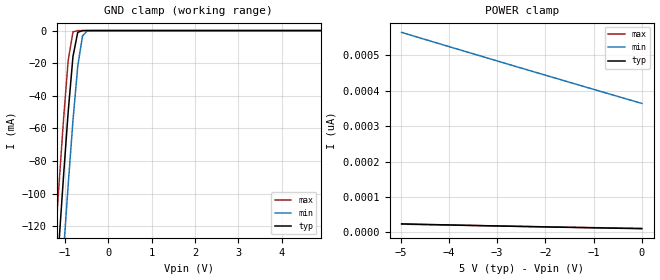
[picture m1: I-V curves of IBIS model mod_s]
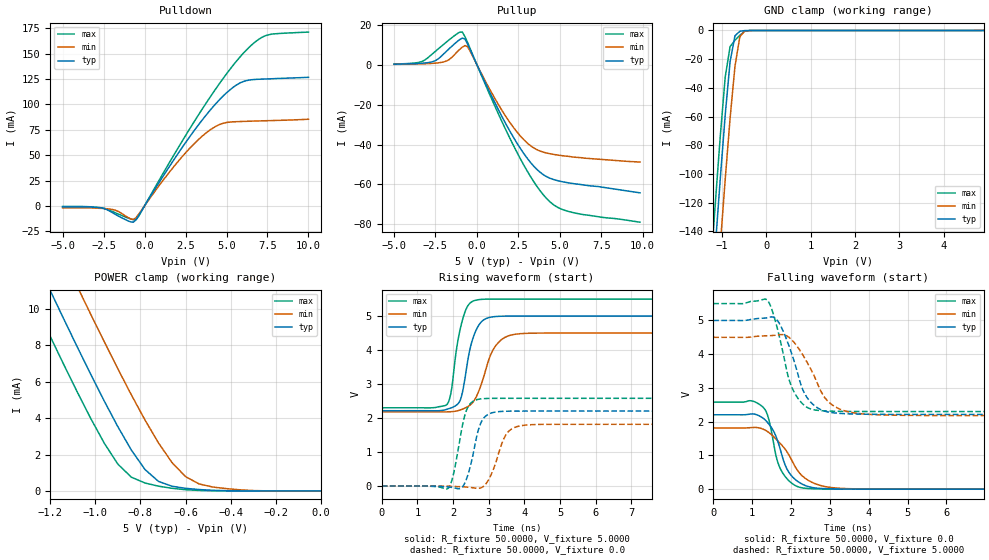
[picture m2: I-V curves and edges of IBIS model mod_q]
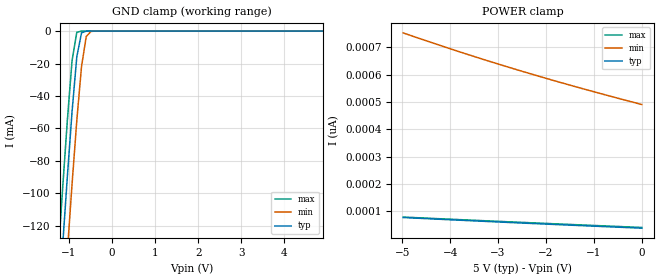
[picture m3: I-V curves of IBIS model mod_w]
| IBIS (I/O, Buffer, Information, Specification) Model, officially
| electronic behavioral standard for Buffer structures of digital pins.
[IBIS ver]  4.0
[File name] m95xxx_g12_tssop8.ibs
[File Rev]  1.0
[Date]   9 Oct 2015
[Source]   CAD & Design Services (Catania) - STMicroelectronics
[Notes]
  (Note1)  This IBIS model includes the TSSOP8 ceramic package parasitic data
  (Note2)  This IBIS model considers: VCC=5.0(TYP), 4.50(MIN), 5.50(MAX)
  (Note3)  This IBIS model has some Notes about the non-monotonicity
   of the I-V curves, but they are not indicative of problems
   inside the model;
[Copyright] (c) 2015 STMicroelectronics
|   Component M95XXX
[Component] M95XXX
[Manufacturer] STMicroelectronics
[Package]
|variable   typ   min   max
R_pkg   0.0   0.0   0.0
L_pkg   0.0H   0.0H   0.0H
C_pkg   0.0F   0.0F   0.0F
[Pin]   signal_name   model_name   R_pin   L_pin   C_pin
1   SN   mod_s   NA   NA   NA
2   Q   mod_q   NA   NA   NA
3   WN   mod_w   NA   NA   NA
4   GND   GND   NA   NA   NA
5   D   mod_s   NA   NA   NA
6   C   mod_s   NA   NA   NA
7   HOLDN   mod_h   NA   NA   NA
8   VCC   POWER   NA   NA   NA
[Package Model]  182696_TSSOP8
[Define Package Model]  182696_TSSOP8
[Manufacturer]  STMicroelectronics
[OEM]  STMicroelectronics
[Description]  8 pin TSSOP package
[Number Of Pins]  8
[Pin Numbers]
|Pin Num   Terminal Name
1   | net1
2   | net2
3   | net3
4   | net4_GND
5   | net5
6   | net6
7   | net7
8   | net8_VDD
[Model Data]
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[End Model Data]
[End Package Model]
| Models and submodels in the file (4): mod_s (Input), mod_q (I/O), mod_w (Input), mod_h (Input)
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|   Model mod_s
[Model]   mod_s
Model_type Input
Vinl   =   1.500V
Vinh   =   3.500V
C_comp   2.119pF   2.024pF   2.323pF
[Temperature Range]   25.0000   0.1050k   -40.0000
[Voltage Range]   5.0000V   4.5000V   5.5000V
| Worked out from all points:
|   GND clamp passes 1 mA (typ) near -0.70 V on its own axis
[GND_clamp]
|Voltage   I(typ)   I(min)   I(max)
-5V       -1.764A    -1.807A    -1.733A
-1.26V    -176.7mA   -223.6mA   -141.2mA
-1.15V    -132.7mA   -179.4mA   -97.27mA
-1.04V    -89.88mA   -136.2mA   -55.14mA
-930mV    -49.58mA   -94.31mA   -18.16mA
-820mV    -15.87mA   -55.06mA   -757uA
-710mV    -1.068mA   -21.8mA    -5.45uA
-600mV    -23.1uA    -3.301mA   -36.27nA
-490mV    -459.2nA   -183.8uA   -242.2pA
4.9V      10.56pA    379.5pA    10.13pA
[POWER_clamp]
|Voltage   I(typ)   I(min)   I(max)
-4.98V    24.27pA    563.8pA    23.46pA
-3.96V    21.17pA    522.2pA    20.77pA
-2.64V    17.45pA    468.9pA    17.5pA
0V        10.79pA    363.7pA    11.44pA
|   Model mod_q
[Model]   mod_q
Model_type I/O
Polarity   Non-Inverting
Enable   Active-Low
Vinl   =   1.500V
Vinh   =   3.500V
Vmeas  =   2.500V
Cref   =   30pF
C_comp   2.793pF   2.547pF   3.063pF
[Temperature Range]  25.0000   0.1050k   -40.0000
[Voltage Range]   5.0000V   4.5000V   5.5000V
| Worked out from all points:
|   slope of the pulldown table from 0 to 0.75 V, typ, clamps not added: 38.4 ohm
|   slope of the pullup table from 0 to 0.75 V, typ, clamps not added: 56.1 ohm
|   GND clamp passes 1 mA (typ) near -0.62 V on its own axis
|   POWER clamp passes 1 mA (typ) near -0.76 V on its own axis
|   rising waveform, R_fixture 50.0000, V_fixture 5.0000: 20-80 % time 324ps typ, 480ps min, 286ps max; typ from 2.21 V to 5 V
|   rising waveform, R_fixture 50.0000, V_fixture 0.0: 20-80 % time 297ps typ, 373ps min, 281ps max; typ from 0 V to 2.21 V
|   falling waveform, R_fixture 50.0000, V_fixture 0.0: 20-80 % time 452ps typ, 681ps min, 339ps max; typ from 2.21 V to 0 V
|   falling waveform, R_fixture 50.0000, V_fixture 5.0000: 20-80 % time 497ps typ, 646ps min, 427ps max; typ from 5 V to 2.21 V
[Pulldown]
|Voltage   I(typ)   I(min)   I(max)
-5V       -1mA       -2mA       -600uA
-2.6V     -2.1mA     -2.5mA     -2mA
-1.8V     -8.2mA     -4.2mA     -6.7mA
-840mV    -15.83mA   -12.84mA   -12.96mA
-520mV    -13.63mA   -11.72mA   -13.73mA
1.4V      35.96mA    30.85mA    39.51mA
3V        73.61mA    60.85mA    82.31mA
4.28V     99.55mA    77.79mA    113.9mA
5.24V     114.8mA    82.7mA     135.3mA
6.2V      123.5mA    83.38mA    153.5mA
7.32V     125.1mA    83.93mA    167.5mA
10V       126.8mA    85.45mA    171.4mA
[Pullup]
|Voltage   I(typ)   I(min)   I(max)
-5V       270uA      190uA      350uA
-3.44V    670uA      405uA      1.305mA
-2.64V    1.605mA    706uA      5.755mA
-1.68V    7.984mA    2.565mA    12.44mA
-880mV    13.35mA    8.83mA     16.36mA
-560mV    10.29mA    8.992mA    11.08mA
1.04V     -18.3mA    -16.27mA   -19.93mA
2.32V     -37.98mA   -32.67mA   -42.33mA
3.28V     -49.41mA   -40.84mA   -56.63mA
4.24V     -56.24mA   -44.29mA   -67.33mA
5.68V     -59.39mA   -46.1mA    -73.85mA
9.84V     -64.2mA    -48.78mA   -78.9mA
[GND_clamp]
|Voltage   I(typ)   I(min)   I(max)
-5V       -1.919A    -1.961A    -1.893A
-1.26V    -197.2mA   -244mA     -167mA
-1.15V    -149.4mA   -196.2mA   -119.1mA
-1.04V    -102.8mA   -149.2mA   -73.18mA
-930mV    -58.88mA   -103.8mA   -32.39mA
-820mV    -21.66mA   -61.22mA   -11.23mA
-710mV    -3.687mA   -24.94mA   -6.819mA
-600mV    -560.4uA   -4.331mA   -3.354mA
-490mV    -78.82uA   -439.8uA   -616.8uA
-380mV    -6.109uA   -68.67uA   -6.344uA
4.9V      210.5pA    105.8uA    176.1pA
[POWER_clamp]
|Voltage   I(typ)   I(min)   I(max)
-4.98V    114.4mA    117.5mA    112.1mA
-1.32V    14.15mA    17.49mA    11.63mA
-1.26V    12.57mA    15.9mA     10.05mA
-1.2V     10.99mA    14.33mA    8.479mA
-1.08V    7.9mA      11.22mA    5.424mA
-1.02V    6.392mA    9.687mA    3.968mA
-960mV    4.924mA    8.178mA    2.612mA
-840mV    2.238mA    5.266mA    752uA
-720mV    522.7uA    2.637mA    261.1uA
-600mV    143uA      786uA      68.21uA
-420mV    12.23uA    128uA      1.15uA
0V        225pA      1.615nA    241.5pA
[Ramp]
| variable   typ   min   max
dV/dt_r  1.3231/0.3352n   1.0895/0.4279n   1.5474/0.3147n
dV/dt_f  1.6706/0.5497n   1.3898/0.7138n   1.9193/0.4691n
R_load = 50.0000
[Rising Waveform]
R_fixture= 50.0000
V_fixture= 5.0000
V_fixture_min= 4.5000
V_fixture_max= 5.5000
|time   V(typ)   V(min)   V(max)
0s        2.215V     2.181V     2.301V
1.845ns   2.264V     2.181V     2.418V
1.935ns   2.293V     2.185V     2.703V
2.115ns   2.395V     2.21V      4.148V
2.265ns   2.761V     2.261V     4.888V
2.475ns   4.029V     2.379V     5.379V
2.655ns   4.602V     2.632V     5.471V
3.135ns   4.98V      4.027V     5.499V
3.735ns   5V         4.463V     5.5V
15ns      5V         4.5V       5.5V
[Rising Waveform]
R_fixture= 50.0000
V_fixture= 0.0
V_fixture_min= 0.0
V_fixture_max= 0.0
|time   V(typ)   V(min)   V(max)
0s        7.297nV    284nV      7.334nV
1.875ns   -26.33mV   -5.976mV   -60.61mV
2.025ns   -53.4mV    -12.66mV   410.9mV
2.325ns   75.33mV    -26.36mV   2.059V
2.475ns   541.6mV    -41.89mV   2.413V
2.745ns   1.763V     -64.96mV   2.557V
3.045ns   2.137V     279.4mV    2.578V
3.495ns   2.2V       1.523V     2.58V
3.915ns   2.204V     1.776V     2.58V
15ns      2.205V     1.815V     2.58V
[Falling Waveform]
R_fixture= 50.0000
V_fixture= 0.0
V_fixture_min= 0.0
V_fixture_max= 0.0
|time   V(typ)   V(min)   V(max)
0s        2.205V     1.815V     2.58V
945ps     2.225V     1.822V     2.623V
1.275ns   2.109V     1.782V     2.435V
1.425ns   1.937V     1.684V     2.086V
1.605ns   1.59V      1.495V     1.043V
1.725ns   1.18V      1.351V     609.1mV
1.935ns   519.9mV    1.037V     263.7mV
2.295ns   145.8mV    389.4mV    37.35mV
3.465ns   3.378mV    15.12mV    583uV
15ns      -6.782nV   272nV      1.021nV
[Falling Waveform]
R_fixture= 50.0000
V_fixture= 5.0000
V_fixture_min= 4.5000
V_fixture_max= 5.5000
|time   V(typ)   V(min)   V(max)
0s        5V         4.5V       5.5V
1.38ns    5.079V     4.546V     5.615V
1.68ns    4.95V      4.573V     4.62V
1.92ns    4.336V     4.523V     3.376V
2.04ns    3.94V      4.402V     2.974V
2.31ns    2.932V     3.967V     2.517V
2.61ns    2.47V      3.321V     2.348V
3.03ns    2.272V     2.525V     2.312V
3.84ns    2.222V     2.231V     2.302V
15ns      2.215V     2.181V     2.301V
|   Model mod_w
[Model]   mod_w
Model_type Input
Vinl   =   1.500V
Vinh   =   3.500V
C_comp   2.119pF   2.024pF   2.323pF
[Temperature Range]  25.0000   0.1050k   -40.0000
[Voltage Range]   5.0000V   4.5000V   5.5000V
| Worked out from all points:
|   GND clamp passes 1 mA (typ) near -0.70 V on its own axis
[GND_clamp]
|Voltage   I(typ)   I(min)   I(max)
-5V       -1.764A    -1.807A    -1.733A
-1.26V    -176.7mA   -223.6mA   -141.2mA
-1.15V    -132.7mA   -179.4mA   -97.27mA
-1.04V    -89.88mA   -136.2mA   -55.14mA
-930mV    -49.58mA   -94.31mA   -18.16mA
-820mV    -15.87mA   -55.06mA   -757uA
-710mV    -1.068mA   -21.8mA    -5.45uA
-600mV    -23.1uA    -3.301mA   -36.27nA
-490mV    -459.2nA   -183.8uA   -242.2pA
4.9V      10.56pA    379.5pA    10.13pA
[POWER_clamp]
|Voltage   I(typ)   I(min)   I(max)
-4.98V    76.74pA    752.7pA    78.35pA
-3.84V    67.2pA     685.5pA    69.26pA
-2.58V    57.11pA    616.4pA    59.5pA
-1.32V    47.46pA    552.6pA    50.01pA
0V        37.74pA    490.4pA    40.3pA
